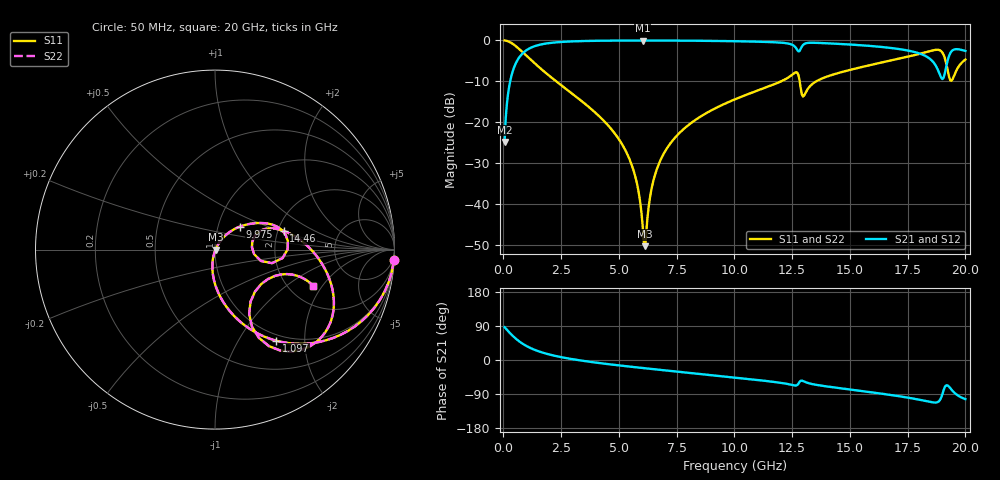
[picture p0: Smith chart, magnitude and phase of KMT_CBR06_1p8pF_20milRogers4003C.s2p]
! Data measured by Modelithics Inc. support@modelithics.com 813-866-6335
! KEMET CBR0603 1.8pF, Pad Width= 0.851mm, Pad Length= 0.64mm, Pad Gap= 0.62mm, 20mil Rogers 4003C substrate Data, January 2022
# hz S ma R 50
! 2 Port Network Data from SP1.SP block
! freq  magS11  angS11  magS21  angS21  magS12  angS12  magS22  angS22
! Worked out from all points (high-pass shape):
!   401 points, 50 MHz to 20 GHz, reference 50 ohm
!   highest |S21| = -0.03 dB at 6.035 GHz (marker M1); lowest = -24.9 dB at 50 MHz (marker M2)
!   |S21| within 3 dB of the highest: 856.6 MHz to 17.92 GHz (17.06 GHz wide, 182 % of centre); 19.36 GHz to end of sweep
!   lowest |S11| = -50.3 dB at 6.135 GHz (marker M3), VSWR 1.01, Z = 50.3 - j0.0146 ohm
!   |S11| at or under -10 dB: 2.283 GHz to 12.02 GHz (9.739 GHz wide, 136 % of centre); 12.83 GHz to 13.54 GHz (719 MHz wide, 5.45 % of centre)
!   |S22| runs from -50.3 to 0.0 dB; largest |S21 - S12| = 0
!   S11 on the Smith chart (normalised r, x): 50 MHz: 1, -33; 1.097 GHz: 0.91, -1.46; 9.975 GHz: 1.27, +0.34; 14.46 GHz: 2.15, +0.53; 20 GHz: 2.68, -1.64
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5e7  0.9984 -3.5  0.05717 86.5  0.05717 86.5  0.9984 -3.5
3.99125e8  0.9085 -26.1  0.4169 63.9  0.4169 63.9  0.9085 -26.1
1.097375e9  0.6107 -56.1  0.7903 33.7  0.7903 33.7  0.6107 -56.1
3.391625e9  0.1806 -91.0  0.9811 -1.7  0.9811 -1.7  0.1806 -91.0
5.33675e9  0.04213 -102.9  0.9962 -16.6  0.9962 -16.6  0.04213 -102.9
5.785625e9  0.01754 -100.4  0.9968 -19.6  0.9968 -19.6  0.01754 -100.4
6.035e9  0.005052 -76.7  0.9969 -21.2  0.9969 -21.2  0.005052 -76.7
6.13475e9  0.003055 -2.7  0.9969 -21.9  0.9969 -21.9  0.003055 -2.7
6.434e9  0.01648 55.9  0.9967 -23.8  0.9967 -23.8  0.01648 55.9
6.73325e9  0.03122 58.8  0.9963 -25.7  0.9963 -25.7  0.03122 58.8
7.880375e9  0.08624 55.0  0.9927 -32.8  0.9927 -32.8  0.08624 55.0
9.975125e9  0.188 42.8  0.9777 -45.9  0.9777 -45.9  0.188 42.8
1.0025e10  0.1905 42.5  0.9772 -46.3  0.9772 -46.3  0.1905 42.5
1.26185e10  0.4031 11.1  0.8374 -67.3  0.8374 -67.3  0.4031 11.1
1.296762e10  0.2063 3.7  0.8778 -55.4  0.8778 -55.4  0.2063 3.7
1.336662e10  0.2921 22.5  0.9359 -63.5  0.9359 -63.5  0.2921 22.5
1.446388e10  0.3968 15.2  0.9086 -73.5  0.9086 -73.5  0.3968 15.2
1.670825e10  0.5632 -3.2  0.8121 -91.8  0.8121 -91.8  0.5632 -3.2
1.850375e10  0.7449 -27.9  0.5825 -111.0  0.5825 -111.0  0.7449 -27.9
1.90025e10  0.7112 -53.0  0.3364 -90.5  0.3364 -90.5  0.7112 -53.0
1.94015e10  0.3211 -36.7  0.7367 -78.5  0.7367 -78.5  0.3211 -36.7
2e10  0.5829 -20.3  0.7445 -103.4  0.7445 -103.4  0.5829 -20.3
